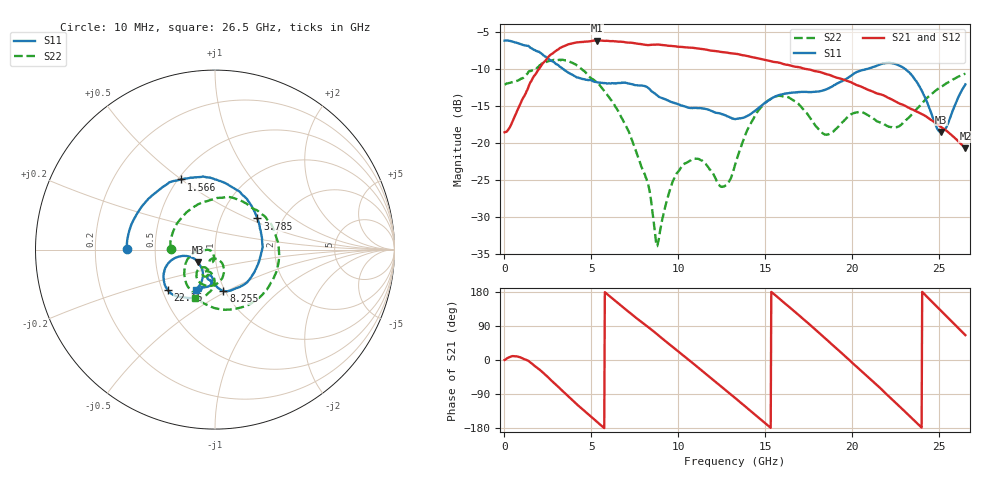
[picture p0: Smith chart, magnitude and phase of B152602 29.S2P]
!  2-Port S-parameters saved by WinCal
! VAR MeasName=S-Parameters (CALIBRATED_DATA) read from VNA (N5242A)
! VAR MeasDate=2016-1-5 16:30:31
! VAR NAME=B152602 29
! VAR FILENAME=B152602 29.S2P
! VAR DATE=2016-1-5 16:30:31
! VAR PHYS_PORTS=1,2
# Hz S DB R 50
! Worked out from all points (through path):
!   801 points, 10 MHz to 26.5 GHz, reference 50 ohm
!   highest |S21| = -6.17 dB at 5.341 GHz (marker M1); lowest = -20.7 dB at 26.5 GHz (marker M2)
!   lowest |S11| = -18.5 dB at 25.08 GHz (marker M3), VSWR 1.27, Z = 41 - j5.88 ohm
!   |S11| at or under -10 dB: 3.352 GHz to 20.88 GHz (17.53 GHz wide, 145 % of centre); 23.02 GHz to end of sweep
!   |S22| runs from -34.0 to -8.8 dB; largest |S21 - S12| = 0.0034
!   S11 on the Smith chart (normalised r, x): 10 MHz: 0.34, +0.00; 1.566 GHz: 0.52, +0.50; 3.785 GHz: 1.49, +0.57; 8.255 GHz: 0.98, -0.48; 22.16 GHz: 0.53, -0.27; 26.5 GHz: 0.73, -0.35
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1e7  -6.17 179.6  -18.59 0.2  -18.56 0.2  -12.14 179.3
1.566288e9  -7.24 115.9  -11.55 -9.1  -11.55 -9.1  -10.22 62.4
2.592775e9  -8.76 76.6  -8.21 -49.2  -8.20 -49.2  -8.92 -3.7
3.784825e9  -10.66 36.2  -6.62 -101.0  -6.63 -101.0  -9.08 -67.8
4.447075e9  -11.36 17.2  -6.37 -128.6  -6.37 -128.5  -10.06 -96.8
5.341112e9  -11.83 -8.1  -6.17 -164.0  -6.17 -164.0  -11.87 -126.7
6.963625e9  -11.88 -48.6  -6.42 133.7  -6.40 133.8  -17.64 -168.7
8.255012e9  -12.56 -78.4  -6.79 87.0  -6.75 87.0  -25.57 -177.8
8.851038e9  -13.74 -87.5  -6.72 65.1  -6.68 65.0  -33.26 -128.3
9.745075e9  -14.61 -94.5  -6.94 31.8  -6.93 31.9  -24.89 -95.4
1.083779e10  -15.30 -99.3  -7.16 -8.7  -7.15 -8.7  -22.21 -107.2
1.249341e10  -16.13 -106.0  -7.73 -70.9  -7.70 -70.9  -25.97 -99.3
1.3255e10  -16.78 -102.9  -7.96 -99.8  -7.94 -99.9  -23.02 -65.6
1.534109e10  -14.03 -97.1  -8.99 179.7  -8.96 179.8  -14.04 -92.5
1.769208e10  -13.13 -110.1  -10.20 87.6  -10.16 87.7  -17.05 -129.9
1.8553e10  -12.72 -109.0  -10.75 52.6  -10.71 52.2  -18.89 -116.7
1.967882e10  -11.32 -111.7  -11.63 6.0  -11.57 5.8  -16.65 -105.3
2.209604e10  -9.20 -138.3  -13.97 -95.9  -13.90 -96.3  -17.85 -110.9
2.216226e10  -9.20 -139.5  -14.04 -98.8  -14.00 -99.2  -17.86 -110.1
2.355299e10  -11.26 -163.5  -15.60 -159.3  -15.60 -159.3  -15.81 -91.8
2.507616e10  -18.54 -143.3  -17.83 131.0  -17.79 130.8  -12.49 -97.0
2.65e10  -12.11 -115.9  -20.75 65.6  -20.71 65.4  -10.65 -112.5
